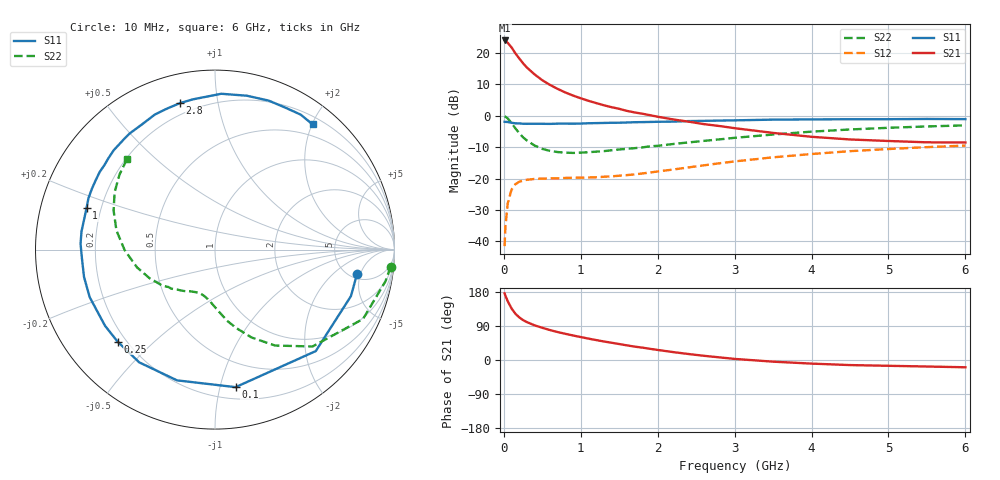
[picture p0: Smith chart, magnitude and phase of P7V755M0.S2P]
! SIEMENS Small Signal Semiconductors
! BFP196
! Si NPN RF Bipolar Junction Transistor in SOT143
! VCE = 0.75 V  IC = 5 mA
! Common Emitter S-Parameters:  May  1996
# GHz  S  MA  R  50
!  f  S11  S21  S12  S22
! GHz  MAG  ANG  MAG  ANG  MAG  ANG  MAG  ANG
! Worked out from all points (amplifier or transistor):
!   36 points, 10 MHz to 6 GHz, reference 50 ohm
!   highest |S21| = 24.0 dB at 10 MHz (marker M1)
!   |S21| within 3 dB of that: start of sweep to 121 MHz
!   unconditionally stable (mu >= 1): 1.075 GHz to end of sweep
!   at 250 MHz: K = 0.27, MSG = 18.7 dB, |S12| = -20.6 dB
!   at 1.4 GHz: K = 1.16, MAG = 8.6 dB, |S12| = -19.3 dB
!   at 6 GHz: K = 1.05, MAG = -0.9 dB, |S12| = -9.5 dB
!   S11 on the Smith chart (normalised r, x): 10 MHz: 5.71, -4.39; 100 MHz: 0.29, -1.12; 250 MHz: 0.17, -0.39; 1 GHz: 0.14, +0.15; 2.8 GHz: 0.14, +0.78; 6 GHz: 0.31, +2.01
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0.01  0.8029 -9.8  15.83 175.9  0.0084 86.8  0.9832 -5.5
0.02  0.8005 -18.9  15.38 169.6  0.0168 80.4  0.9663 -10.5
0.05  0.7968 -45.2  14.55 155.5  0.0401 67.0  0.9109 -25.1
0.1  0.7749 -81.5  12.28 136.1  0.0669 50.5  0.766 -44.8
0.15  0.7586 -106.2  9.873 122.2  0.0813 39.4  0.6311 -57.9
0.2  0.7569 -123.9  8.211 112.6  0.0889 32.3  0.5304 -67.4
0.25  0.7466 -136.6  6.842 105.3  0.093 27.4  0.4539 -74.7
0.3  0.7454 -145.3  5.858 100.0  0.0957 24.3  0.4043 -80.1
0.4  0.7468 -159.2  4.558 91.5  0.0988 20.3  0.3361 -87.8
0.5  0.7455 -168.2  3.683 85.0  0.1 18.3  0.2973 -94.0
0.6  0.743 -176.2  3.1 79.0  0.1007 17.6  0.276 -99.1
0.7  0.7498 177.5  2.679 73.7  0.101 17.3  0.2646 -103.4
0.8  0.7506 172.3  2.349 69.1  0.1025 17.3  0.2592 -107.1
1  0.7521 162.1  1.9 60.5  0.1034 18.8  0.2591 -113.3
1.1  0.7608 158.0  1.732 56.4  0.1041 20.1  0.2632 -116.5
1.6  0.7821 139.4  1.197 38.6  0.1137 26.6  0.2981 -130.3
2.2  0.8074 120.3  0.875 20.9  0.1394 32.2  0.3554 -145.5
2.8  0.839 103.4  0.688 7.0  0.1753 32.0  0.4208 -162.3
3.5  0.8689 87.7  0.534 -4.4  0.2182 26.5  0.5031 -179.6
4.5  0.8824 70.2  0.42 -13.4  0.2734 15.6  0.6055 158.9
5.5  0.8907 57.6  0.378 -17.2  0.3171 4.0  0.6769 141.8
6  0.8845 52.0  0.376 -19.2  0.3355 -2.3  0.7035 134.1
